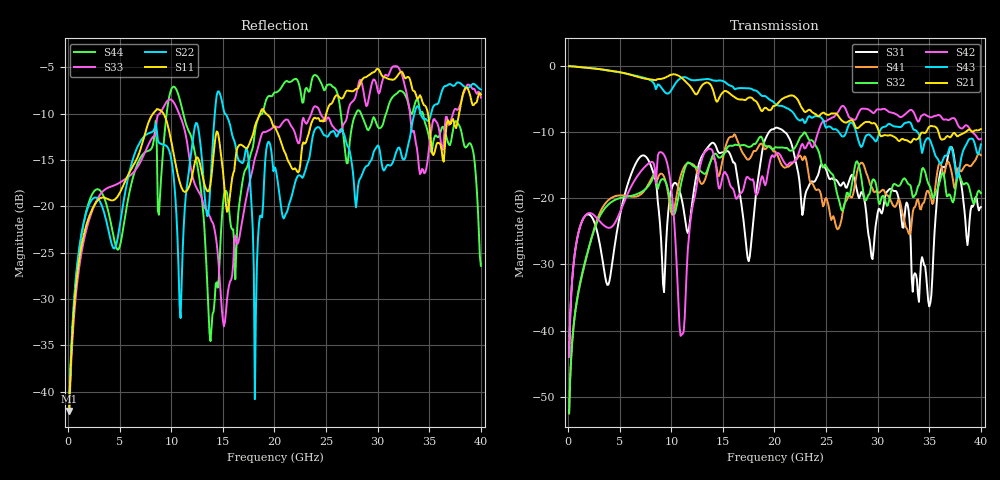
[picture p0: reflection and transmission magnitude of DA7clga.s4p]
! ADC12DJ3200QML-SP
! 196-pin ZMX package
! CLGA Ceramic Package without columns (ceramic land grid array)
! Texas Instruments 4/21/2021
! Single-ended  S-parameters
! PORT#  PORT_NAME  NET_NAME
! PORT1:  DAxN.DIEBUMP DAxN
! PORT2:  DAxN.BGA  DAxN
! PORT3:  DAxP.DIEBUMP DAxP
! PORT4:  DAxP.BGA  DAxP
! Touchstone Ver. 1.0
! Number of ports is 4
# Hz	S	MA	R	50.000000
! SCATTERING PARAMETERS  :
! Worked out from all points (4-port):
!   400 points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, 100 MHz to 40 GHz, reference 50 ohm
!   strongest paths, dB at 100 MHz, 10.1 GHz, 20.1 GHz, 30.1 GHz, 40 GHz:
!     S21: -0.1, -1.3, -6.0, -9.9, -9.6
!     S43: -0.1, -3.4, -5.8, -10.3, -11.9
!     S42: -43.9, -20.1, -13.4, -6.6, -11.0
!     S32: -52.5, -22.0, -12.3, -20.7, -19.2
!     S41: -52.5, -22.5, -13.0, -19.2, -13.5
!     S31: -43.9, -18.2, -9.4, -21.6, -21.3
!   lowest |S11| = -42.0 dB at 100 MHz (marker M1), VSWR 1.02, Z = 50.6 - j0.464 ohm
!   |S11| at or under -10 dB: start of sweep to 8.242 GHz; 9.235 GHz to 18.6 GHz (9.365 GHz wide, 67.3 % of centre); 19.17 GHz to 25.02 GHz (5.849 GHz wide, 26.5 % of centre)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
1e8  0.0079 -35.5  0.993 -3.4  0.006383 76.8  0.002378 -119.6
     0.993 -3.4  0.00815 -35.7  0.002378 -119.5  0.006361 77.1
     0.006383 76.8  0.002378 -119.5  0.00766 -32.6  0.993 -3.4
     0.002378 -119.6  0.006361 77.1  0.993 -3.4  0.007964 -32.8
5.3e9  0.1278 -15.0  0.8852 -173.2  0.09318 78.0  0.1049 66.3
       0.8852 -173.2  0.09999 -108.2  0.1014 68.1  0.08852 45.4
       0.09318 78.0  0.1014 68.1  0.1374 4.9  0.8835 -172.5
       0.1049 66.3  0.08852 45.4  0.8835 -172.5  0.07366 -116.4
1.08e10  0.1363 108.5  0.8325 11.1  0.1137 7.6  0.1375 -86.5
         0.8325 11.1  0.02954 57.7  0.1131 -82.3  0.01076 145.8
         0.1137 7.6  0.1131 -82.3  0.3114 75.3  0.7944 29.9
         0.1375 -86.5  0.01076 145.8  0.7944 29.9  0.3807 167.2
1.38e10  0.1323 -58.0  0.719 -84.7  0.2562 12.6  0.1888 166.2
         0.719 -84.7  0.1337 -106.3  0.1888 170.1  0.2356 -0.4
         0.2562 12.6  0.1888 170.1  0.08651 -65.4  0.787 -73.1
         0.1888 166.2  0.2356 -0.4  0.787 -73.1  0.01876 -32.4
1.81e10  0.27 160.1  0.546 149.6  0.08972 103.6  0.2268 2.6
         0.546 149.6  0.00913 133.2  0.256 8.8  0.1146 100.0
         0.08972 103.6  0.256 8.8  0.1812 -170.0  0.6517 145.8
         0.2268 2.6  0.1146 100.0  0.6517 145.8  0.2506 -84.6
2.12e10  0.1828 -6.1  0.5845 66.1  0.3053 -66.6  0.1729 -115.6
         0.5845 66.1  0.09296 -146.8  0.2397 -103.1  0.177 65.5
         0.3053 -66.6  0.2397 -103.1  0.2934 6.9  0.4772 49.4
         0.1729 -115.6  0.177 65.5  0.4772 49.4  0.4746 -140.7
4e10  0.401 146.3  0.3324 -119.2  0.08584 -5.6  0.2113 -14.3
      0.3324 -119.2  0.4266 160.4  0.1092 49.5  0.2805 -63.3
      0.08584 -5.6  0.1092 49.5  0.3857 -157.7  0.255 -109.4
      0.2113 -14.3  0.2805 -63.3  0.255 -109.4  0.0478 134.8
